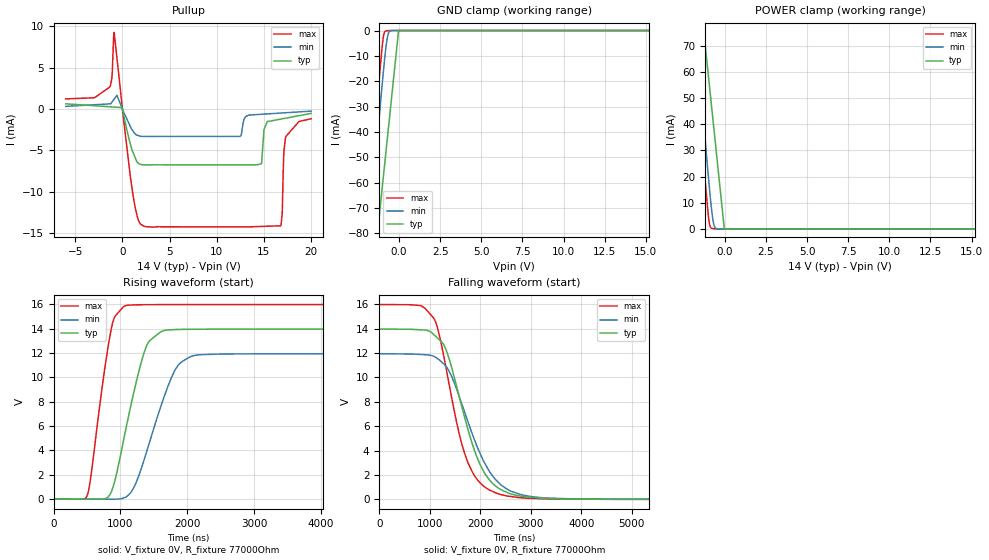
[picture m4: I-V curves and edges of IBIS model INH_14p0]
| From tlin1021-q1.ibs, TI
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|   INH_2021
[Model]   INH_14p0
Model_type   Open_source
Polarity   Non-Inverting
Vmeas = 7
Vref = 7
Cref = 2pF
Rref = 77000
|   typ   min   max
C_comp   1.675pF   1.6pF   1.754pF
[Voltage Range]   14   12   16
[Temperature Range]   25   165   -55
[Pullup Reference]   14   12   16
[Pulldown Reference]   0   0   0
[Power Clamp Reference]   14   12   16
[GND Clamp Reference]   0   0   0
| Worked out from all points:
|   slope of the pullup table from 0 to 2.1 V, typ, clamps not added: 311 ohm
|   GND clamp passes 1 mA (typ) near -0.04 V on its own axis
|   POWER clamp passes 1 mA (typ) near -0.04 V on its own axis
|   falling waveform, V_fixture 0V, R_fixture 77000Ohm: 20-80 % time 596ns typ, 681ns min, 513ns max; typ from 14 V to 0 V
|   rising waveform, V_fixture 0V, R_fixture 77000Ohm: 20-80 % time 338ns typ, 428ns min, 234ns max; typ from 0 V to 14 V
[GND Clamp]
|   Voltage   I(typ)   I(min)   I(max)
-6V       -446mA     -447.3mA   -446.1mA
-2.075V   -127.8mA   -103mA     -89.37mA
-1.732V   -106.4mA   -75.53mA   -61.01mA
-1.266V   -77.27mA   -39.17mA   -23.9mA
-1.126V   -68.56mA   -28.68mA   -13.41mA
-980.8mV  -59.5mA    -18.36mA   -3.89mA
-906.5mV  -54.86mA   -13.28mA   -1.067mA
-810.3mV  -48.86mA   -7.47mA    -254.7uA
-696.2mV  -41.75mA   -2.364mA   -73.43uA
-587.9mV  -34.99mA   -366.4uA   -9.84uA
-26.96mV  0A         0A         0A
20V       0A         0A         0A
[Pullup]
|   Voltage   I(typ)   I(min)   I(max)
-6V       616.7uA    307.5uA    1.21mA
-1.359V   257.2uA    606.9uA    2.633mA
-1.126V   239.2uA    797.2uA    3.636mA
-874mV    219.7uA    1.198mA    9.27mA
-26.96mV  154.1uA    82.54uA    305.3uA
1.109V    -5.228mA   -2.674mA   -10.33mA
2.511V    -6.776mA   -3.336mA   -14.26mA
14.73V    -6.651mA   -651uA     -14.23mA
15.35V    -1.539mA   -606.3uA   -14.2mA
16.76V    -1.238mA   -504.1uA   -14.15mA
17.28V    -1.127mA   -466.6uA   -3.477mA
20V       -547.3uA   -269.7uA   -1.189mA
[POWER Clamp]
|   Voltage   I(typ)   I(min)   I(max)
-6V       447.1mA    448.6mA    447mA
-1.917V   114.2mA    91.4mA     77.04mA
-1.718V   102.2mA    75.41mA    60.56mA
-1.266V   74.84mA    39.96mA    24.38mA
-1.126V   66.41mA    29.4mA     13.82mA
-980.8mV  57.63mA    19mA       4.211mA
-906.5mV  53.14mA    13.88mA    1.214mA
-810.3mV  47.33mA    7.99mA     280.5uA
-696.2mV  40.44mA    2.678mA    127.5uA
-587.9mV  33.89mA    411.7uA    2.422uA
-26.96mV  0A         0A         0A
20V       0A         0A         0A
[Ramp]
R_load = 77000
|   typ   min   max
dV/dt_r   8.38087/3.3827e-07   7.16787/4.27607e-07   9.58844/2.33985e-07
dV/dt_f   8.38087/5.96252e-07   7.16787/6.81077e-07   9.58844/5.13154e-07
[Falling Waveform]
V_fixture = 0V
V_fixture_min = 0V
V_fixture_max = 0V
R_fixture = 77000Ohm
C_fixture = 0F
|   Time   V(typ)   V(min)   V(max)
0s        13.97V     11.95V     15.98V
821.5ns   13.9V      11.88V     15.89V
1.071us   13.55V     11.74V     14.89V
1.322us   12.26V     10.89V     10.75V
1.582us   8.446V     8.438V     5.386V
1.754us   5.745V     6.375V     3.012V
1.984us   2.96V      3.872V     1.407V
2.324us   1.016V     1.519V     492.7mV
3.287us   70.99mV    108.8mV    39.5mV
9.9us     7.126uV    31.84uV    15.21uV
[Rising Waveform]
V_fixture = 0V
V_fixture_min = 0V
V_fixture_max = 0V
R_fixture = 77000Ohm
C_fixture = 0F
|   Time   V(typ)   V(min)   V(max)
0s        8.018uV    32.29uV    15.49uV
507.5ns   -8.389mV   -5.248mV   364.6mV
864.5ns   599.4mV    -5.604mV   14V
908.1ns   1.326V     -635.3uV   14.88V
1.071us   5.454V     145.8mV    15.87V
1.238us   9.619V     1.377V     15.96V
1.427us   12.93V     4.499V     15.97V
1.823us   13.92V     10.65V     15.97V
2.112us   13.95V     11.8V      15.98V
9.9us     13.97V     11.95V     15.98V
